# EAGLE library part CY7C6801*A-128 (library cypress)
EZ-USB FX2LP (TM) USB Microcontroller Source: http://www.cypress.com .. cy7c68013a_5.pdf
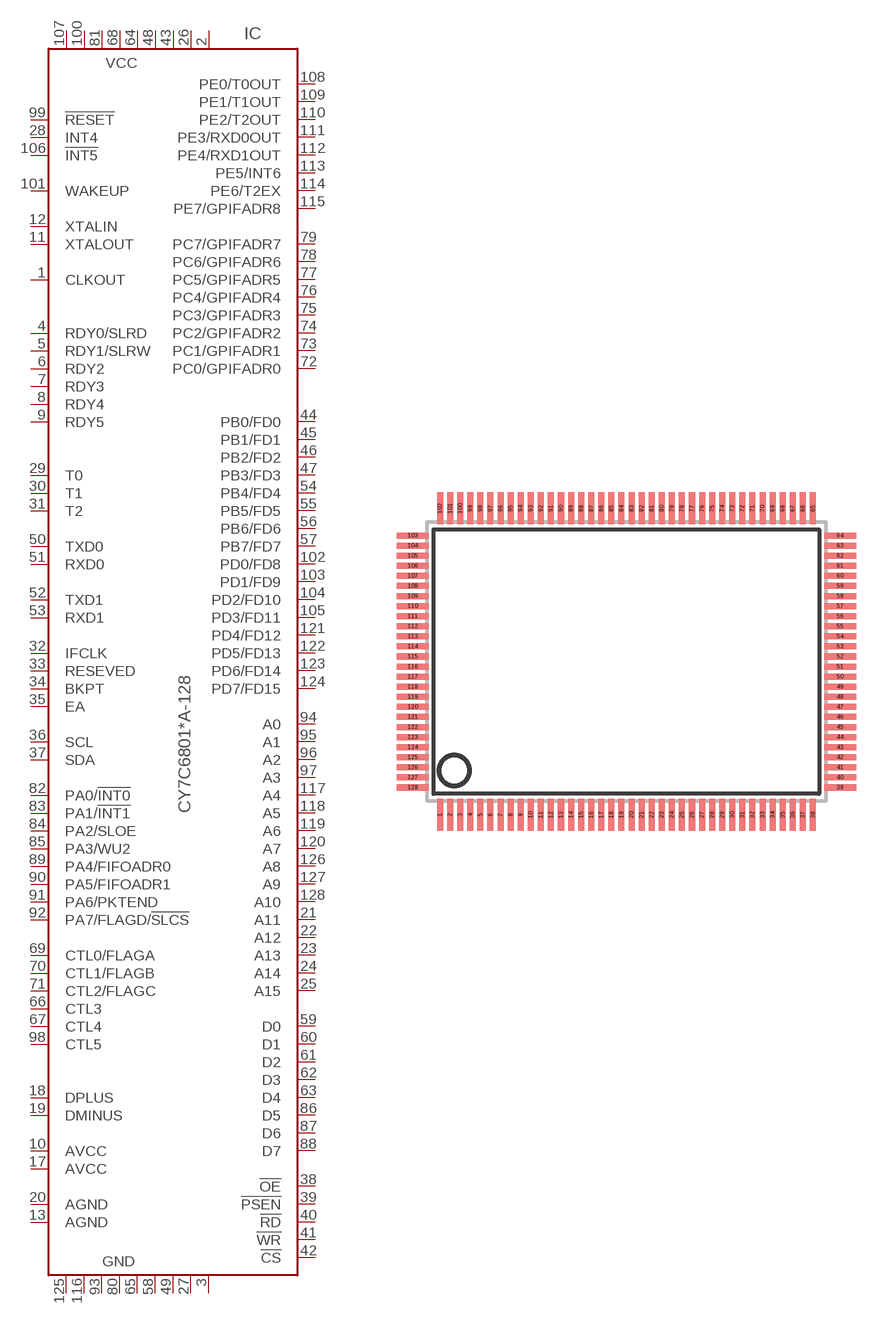
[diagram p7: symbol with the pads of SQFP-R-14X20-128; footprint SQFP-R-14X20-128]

Designator prefix IC

## CY7C68013A-128AXC (MF: CYPRESS SEMICONDUCTOR CORPORAT; MPN: CY7C68013A-128AXC; OC_FARNELL: 1269131; OC_NEWARK: 19M7108), CY7C68014A-128AXC (MPN: CY7C68014A-128AXC; OC_FARNELL: 1269137; OC_NEWARK: 23M5563)  [SQFP-R-14X20-128]
1  CLKOUT  in
2  VCC  in
3  GND  in
4  RDY0/SLRD  in
5  RDY1/SLRW  in
6  RDY2  in
7  RDY3  in
8  RDY4  in
9  RDY5  in
10  AVCC  in
11  XTALOUT  in
12  XTALIN  in
13  AGND  in
17  AVCC  in
18  DPLUS
19  DMINUS
20  AGND  in
21  A11  out
22  A12  out
23  A13  out
24  A14  out
25  A15  out
26  VCC  in
27  GND  in
28  INT4  out
29  T0  out
30  T1  out
31  T2  out
32  IFCLK
33  RESEVED  in
34  BKPT  out
35  EA  in
36  SCL  out
37  SDA
38  !OE  out
39  !PSEN  out
40  !RD  out
41  !WR  out
42  !CS  out
43  VCC  in
44  PB0/FD0
45  PB1/FD1
46  PB2/FD2
47  PB3/FD3
48  VCC  in
49  GND  in
50  TXD0  in
51  RXD0  out
52  TXD1  in
53  RXD1  out
54  PB4/FD4
55  PB5/FD5
56  PB6/FD6
57  PB7/FD7
58  GND  in
59  D0  in
60  D1  in
61  D2  in
62  D3  in
63  D4  in
64  VCC  in
65  GND  in
66  CTL3  in
67  CTL4  in
68  VCC  in
69  CTL0/FLAGA  out
70  CTL1/FLAGB  out
71  CTL2/FLAGC  out
72  PC0/GPIFADR0
73  PC1/GPIFADR1
74  PC2/GPIFADR2
75  PC3/GPIFADR3
76  PC4/GPIFADR4
77  PC5/GPIFADR5
78  PC6/GPIFADR6
79  PC7/GPIFADR7
80  GND  in
81  VCC  in
82  PA0/!INT0
83  PA1/!INT1
84  PA2/SLOE
85  PA3/WU2
86  D5  in
87  D6  in
88  D7  in
89  PA4/FIFOADR0
90  PA5/FIFOADR1
91  PA6/PKTEND
92  PA7/FLAGD/!SLCS
93  GND  in
94  A0  out
95  A1  out
96  A2  out
97  A3  out
98  CTL5
99  !RESET
100  VCC  in
101  WAKEUP  in
102  PD0/FD8
103  PD1/FD9
104  PD2/FD10
105  PD3/FD11
106  !INT5  out
107  VCC  in
108  PE0/T0OUT
109  PE1/T1OUT
110  PE2/T2OUT
111  PE3/RXD0OUT
112  PE4/RXD1OUT
113  PE5/INT6
114  PE6/T2EX
115  PE7/GPIFADR8
116  GND  in
117  A4  out
118  A5  out
119  A6  out
120  A7  out
121  PD4/FD12
122  PD5/FD13
123  PD6/FD14
124  PD7/FD15
125  GND  in
126  A8  out
127  A9  out
128  A10  out

## CY7C68013A-128AXI (MPN: CY7C68013A-128AXI; OC_FARNELL: 1761052; OC_NEWARK: 19M7109)  [SQFP-R-14X20-128]
Pads as for SQFP-R-14X20-128

## Footprint SQFP-R-14X20-128 (pad centres in mm)
QFP128 shrink quad flat pack, rectangle
smd 0.3 x 1.6: 1 -9.25,-7.6; 2 -8.75,-7.6; 3 -8.25,-7.6; 4 -7.75,-7.6; 5 -7.25,-7.6; 6 -6.75,-7.6; 7 -6.25,-7.6; 8 -5.75,-7.6; 9 -5.25,-7.6; 10 -4.75,-7.6; 11 -4.25,-7.6; 12 -3.75,-7.6; 13 -3.25,-7.6; 14 -2.75,-7.6; 15 -2.25,-7.6; 16 -1.75,-7.6; 17 -1.25,-7.6; 18 -0.75,-7.6; 19 -0.25,-7.6; 20 0.25,-7.6; 21 0.75,-7.6; 22 1.25,-7.6; 23 1.75,-7.6; 24 2.25,-7.6; 25 2.75,-7.6; 26 3.25,-7.6; 27 3.75,-7.6; 28 4.25,-7.6; 29 4.75,-7.6; 30 5.25,-7.6; 31 5.75,-7.6; 32 6.25,-7.6; 33 6.75,-7.6; 34 7.25,-7.6; 35 7.75,-7.6; 36 8.25,-7.6; 37 8.75,-7.6; 38 9.25,-7.6; 65 9.25,7.6; 66 8.75,7.6; 67 8.25,7.6; 68 7.75,7.6; 69 7.25,7.6; 70 6.75,7.6; 71 6.25,7.6; 72 5.75,7.6; 73 5.25,7.6; 74 4.75,7.6; 75 4.25,7.6; 76 3.75,7.6; 77 3.25,7.6; 78 2.75,7.6; 79 2.25,7.6; 80 1.75,7.6; 81 1.25,7.6; 82 0.75,7.6; 83 0.25,7.6; 84 -0.25,7.6; 85 -0.75,7.6; 86 -1.25,7.6; 87 -1.75,7.6; 88 -2.25,7.6; 89 -2.75,7.6; 90 -3.25,7.6; 91 -3.75,7.6; 92 -4.25,7.6; 93 -4.75,7.6; 94 -5.25,7.6; 95 -5.75,7.6; 96 -6.25,7.6; 97 -6.75,7.6; 98 -7.25,7.6; 99 -7.75,7.6; 100 -8.25,7.6; 101 -8.75,7.6; 102 -9.25,7.6
smd 1.6 x 0.3: 39 10.6,-6.25; 40 10.6,-5.75; 41 10.6,-5.25; 42 10.6,-4.75; 43 10.6,-4.25; 44 10.6,-3.75; 45 10.6,-3.25; 46 10.6,-2.75; 47 10.6,-2.25; 48 10.6,-1.75; 49 10.6,-1.25; 50 10.6,-0.75; 51 10.6,-0.25; 52 10.6,0.25; 53 10.6,0.75; 54 10.6,1.25; 55 10.6,1.75; 56 10.6,2.25; 57 10.6,2.75; 58 10.6,3.25; 59 10.6,3.75; 60 10.6,4.25; 61 10.6,4.75; 62 10.6,5.25; 63 10.6,5.75; 64 10.6,6.25; 103 -10.6,6.25; 104 -10.6,5.75; 105 -10.6,5.25; 106 -10.6,4.75; 107 -10.6,4.25; 108 -10.6,3.75; 109 -10.6,3.25; 110 -10.6,2.75; 111 -10.6,2.25; 112 -10.6,1.75; 113 -10.6,1.25; 114 -10.6,0.75; 115 -10.6,0.25; 116 -10.6,-0.25; 117 -10.6,-0.75; 118 -10.6,-1.25; 119 -10.6,-1.75; 120 -10.6,-2.25; 121 -10.6,-2.75; 122 -10.6,-3.25; 123 -10.6,-3.75; 124 -10.6,-4.25; 125 -10.6,-4.75; 126 -10.6,-5.25; 127 -10.6,-5.75; 128 -10.6,-6.25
